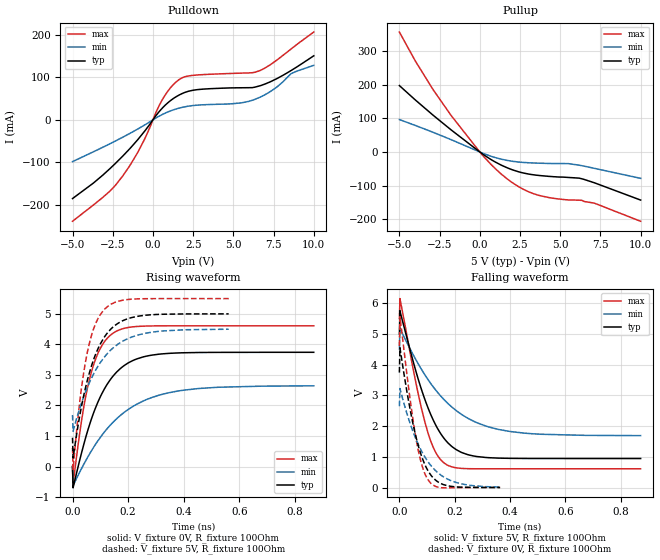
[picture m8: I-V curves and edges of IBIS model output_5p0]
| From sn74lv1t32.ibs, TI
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|   output_5p0 Model
[Model]   output_5p0
Model_type   Output
Polarity   Inverting
Vmeas = 2.5
Vref = 0
Cref = 30pF
Rref = 100
|   typ   min   max
|   (nom PVT)   (fast PVT)   (slow PVT)
C_comp   1.702e-12   1.593e-12   1.738e-12
| Where nom  PVT is Nominal Process, 5V, 40C
|   Fast PVT is Strong Process,  5.5V, -40C
|   Slow PVT is Weak Process,   4.5V, 140C
[Voltage Range]   5   4.5   5.5
|Junction Temperature
[Temperature Range]   40   140   -40
[Pullup Reference]   5   4.5   5.5
[Pulldown Reference]   0   0   0
[Power Clamp Reference]   5   4.5   5.5
[GND Clamp Reference]   0   0   0
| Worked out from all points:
|   slope of the pulldown table from 0 to 0.75 V, typ, clamps not added: 22.1 ohm
|   slope of the pullup table from 0 to 0.75 V, typ, clamps not added: 31.1 ohm
|   falling waveform, V_fixture 5V, R_fixture 100Ohm: 20-80 % time 102ps typ, 174ps min, 74.4ps max; typ from 5 V to 0.944 V
|   rising waveform, V_fixture 0V, R_fixture 100Ohm: 20-80 % time 107ps typ, 178ps min, 67.2ps max; typ from 0 V to 3.74 V
|   rising waveform, V_fixture 5V, R_fixture 100Ohm: 20-80 % time 83.3ps typ, 114ps min, 56.8ps max; typ from 0.943 V to 5 V
|   falling waveform, V_fixture 0V, R_fixture 100Ohm: 20-80 % time 62.3ps typ, 94.4ps min, 48.4ps max; typ from 3.74 V to 0.001 V
[Pulldown]
|   Voltage   I(typ)   I(min)   I(max)
-5V       -184.7mA   -97.99mA   -237.9mA
-2.679V   -114.6mA   -56.15mA   -167.3mA
-1.876V   -85.04mA   -40.68mA   -131.6mA
-913.5mV  -45.17mA   -20.87mA   -74.2mA
604.5mV   28.44mA    12.97mA    48.67mA
1.595V    57.59mA    27.17mA    93.65mA
2.78V     70.99mA    34.61mA    105.4mA
5.49V     75.29mA    39.79mA    109.7mA
6.654V    79.93mA    53.08mA    115.7mA
7.678V    96.21mA    76.28mA    139.5mA
8.599V    115.9mA    108.6mA    166.5mA
10V       150.3mA    127.9mA    206mA
[Pullup]
|   Voltage   I(typ)   I(min)   I(max)
-5V       197.7mA    96.51mA    357.3mA
-4.01V    155mA      79.05mA    271.1mA
-2.94V    111mA      59.21mA    188.4mA
-1.788V   65.93mA    36.74mA    109mA
224.5mV   -7.768mA   -4.512mA   -12.57mA
1.677V    -46.67mA   -24.92mA   -79.32mA
2.711V    -62.73mA   -31.25mA   -111.3mA
3.696V    -70.14mA   -33.47mA   -129.7mA
4.894V    -74.65mA   -34.51mA   -140mA
6.181V    -78.01mA   -39.42mA   -143.6mA
7.105V    -91.56mA   -48.63mA   -152.3mA
10V       -143.3mA   -78.62mA   -206.5mA
[Ramp]
R_load = 100
|   typ   min   max
dV/dt_r   2.2447/1.0744e-10   1.58641/1.77989e-10   2.76554/6.71679e-11
dV/dt_f   2.43368/1.01975e-10   1.68672/1.74302e-10   2.93426/7.43059e-11
[Falling Waveform]
V_fixture = 5V
V_fixture_min = 4.5V
V_fixture_max = 5.5V
R_fixture = 100Ohm
|   Time   V(typ)   V(min)   V(max)
0s        5V         4.5V       5.5V
2ps       5.758V     5.184V     6.15V
64ps      3.652V     4.09V      3.22V
106ps     2.536V     3.48V      1.703V
136ps     1.954V     3.12V      1.068V
170ps     1.507V     2.783V     746.6mV
206ps     1.23V      2.5V       640.1mV
250ps     1.063V     2.241V     612.5mV
402ps     949.2mV    1.821V     609.6mV
872ps     943.9mV    1.689V     609.6mV
[Rising Waveform]
V_fixture = 0V
V_fixture_min = 0V
V_fixture_max = 0V
R_fixture = 100Ohm
|   Time   V(typ)   V(min)   V(max)
0s        608.5pV    5.18nV     1.328nV
2ps       -697.3mV   -626.3mV   -587.7mV
24ps      140.5mV    -218.3mV   971.9mV
40ps      705mV      64mV       1.92V
74ps      1.711V     602mV      3.281V
112ps     2.496V     1.099V     4.052V
156ps     3.068V     1.542V     4.424V
232ps     3.527V     2.045V     4.587V
382ps     3.722V     2.477V     4.609V
868ps     3.741V     2.644V     4.609V
[Rising Waveform]
V_fixture = 5V
V_fixture_min = 4.5V
V_fixture_max = 5.5V
R_fixture = 100Ohm
|   Time   V(typ)   V(min)   V(max)
0s        943.3mV    1.689V     608.4mV
2ps       277.6mV    1.154V     -93.67mV
28ps      1.762V     1.964V     2.268V
42ps      2.393V     2.328V     3.171V
58ps      2.983V     2.689V     3.934V
88ps      3.782V     3.231V     4.779V
118ps     4.285V     3.623V     5.177V
166ps     4.704V     4.023V     5.416V
248ps     4.939V     4.336V     5.495V
562ps     5V         4.498V     5.5V
[Falling Waveform]
V_fixture = 0V
V_fixture_min = 0V
V_fixture_max = 0V
R_fixture = 100Ohm
|   Time   V(typ)   V(min)   V(max)
0s        3.743V     2.645V     4.613V
2ps       4.55V      3.225V     5.555V
36ps      2.677V     2.16V      3.062V
62ps      1.577V     1.532V     1.495V
84ps      925.7mV    1.12V      652.2mV
96ps      671.2mV    938.3mV    372mV
110ps     452.9mV    758.3mV    173.2mV
144ps     157.2mV    444.8mV    5.816mV
206ps     19.37mV    162mV      -3.947mV
364ps     908.6uV    12.11mV    37.29uV
